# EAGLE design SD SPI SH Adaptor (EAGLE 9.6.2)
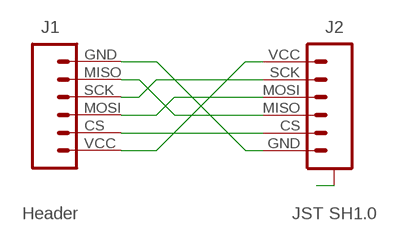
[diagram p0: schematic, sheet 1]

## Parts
J1  Header  HEADER-1X6-SD-SPI  [CONN_06-SD-SPI]
J2  JST SH1.0  JST-SH1.0-6-SMD-HORIZONTAL-SPI  [JST-SH1.0-6-HORIZONTAL-SPI]

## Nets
A: J2.A@1(A) J2.A@6(A)
N$1: J1.GND J2.GND
N$2: J1.VCC J2.VCC
N$3: J1.MISO J2.MISO
N$4: J1.MOSI J2.MOSI
N$5: J1.SCK J2.SCK
N$6: J1.CS J2.CS

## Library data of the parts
J1 = digitalconcepts:HEADER-1X6-SD-SPI: Single Row 6-Pin Header for SD Card Reader SPI Interface
J2 = digitalconcepts:JST-SH1.0-6-SMD-HORIZONTAL-SPI: JST SH1.0 6P SMD SPI horizontal connector

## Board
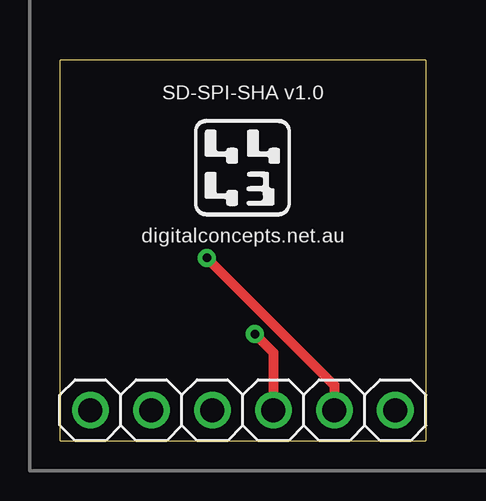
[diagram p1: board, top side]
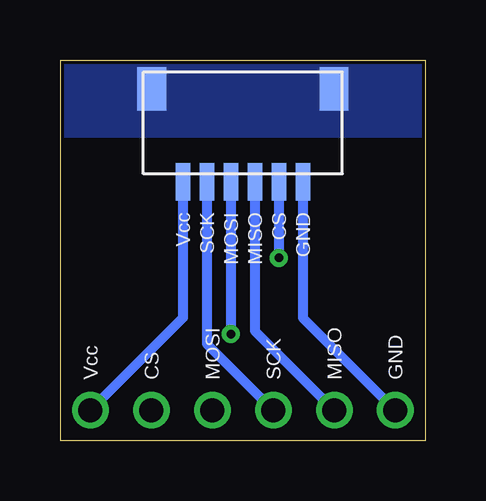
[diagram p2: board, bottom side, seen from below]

Size 15.24 x 15.88 mm. Coordinates in mm from the lower left corner, seen from the top.
Outline: 0,0 15.24,0 15.24,15.88 0,15.88 0,0
Copper layers (1*16): Top 0.035mm / dielectric 1.5mm / Bottom 0.035mm
Design rules "default *": minimum track width 6mil, minimum drill 0.35mm, track to track 6mil, track to pad 6mil, pad to pad 6mil, via to via 6mil, smd to smd 6mil, copper to edge 6mil, drill to drill 6mil, minimum pad ring 10mil, minimum via ring 8mil, stop-mask expansion 4mil, vias tented up to drill 0mil, thermal gap 10mil

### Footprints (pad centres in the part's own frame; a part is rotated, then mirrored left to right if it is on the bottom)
CONN_06-SD-SPI = drill 1 pad 1.524: CS 2.54,0; GND 12.7,0; MISO 10.16,0; MOSI 5.08,0; SCK 7.62,0; VCC 0,0
JST-SH1.0-6-HORIZONTAL-SPI = smd 1.2 x 1.8: A@1 -3.8,-1.335; A@6 3.8,-1.335 | smd 0.6 x 1.55: CS -1.5,2.54; GND -2.5,2.54; MISO -0.5,2.54; MOSI 0.5,2.54; SCK 1.5,2.54; VCC 2.5,2.54

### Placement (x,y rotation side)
J1  13.97,1.27 180 top
J2  7.62,13.34 180 bottom

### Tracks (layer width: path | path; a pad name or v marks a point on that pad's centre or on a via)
A
  pour Bottom (no thermals): 15.24,15.88 15.24,12.7 0,12.7 0,15.88
N$1
  Bottom 0.406: J2.GND 5.12,7.03 5.12,5.12 J1.GND
N$2
  Bottom 0.406: J2.VCC 10.12,5.12 J1.VCC
N$3
  Bottom 0.406: J1.MISO 7.12,4.58 J2.MISO
N$4  (via drill 0.35)
  Top 0.406: v8.12,4.45 8.89,3.68 J1.MOSI
  Bottom 0.406: J2.MOSI v8.12,4.45
N$5
  Bottom 0.406: J2.SCK 9.12,4.04 J1.SCK
N$6  (via drill 0.35)
  Top 0.406: v6.12,7.62 11.43,2.31 J1.CS
  Bottom 0.406: J2.CS v6.12,7.62

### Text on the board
tPlace: SD-SPI-SHA v1.0 | digitalconcepts.net.au
bNames: GND | CS | MISO | MOSI | SCK | Vcc | GND | MISO | SCK | MOSI | CS | Vcc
